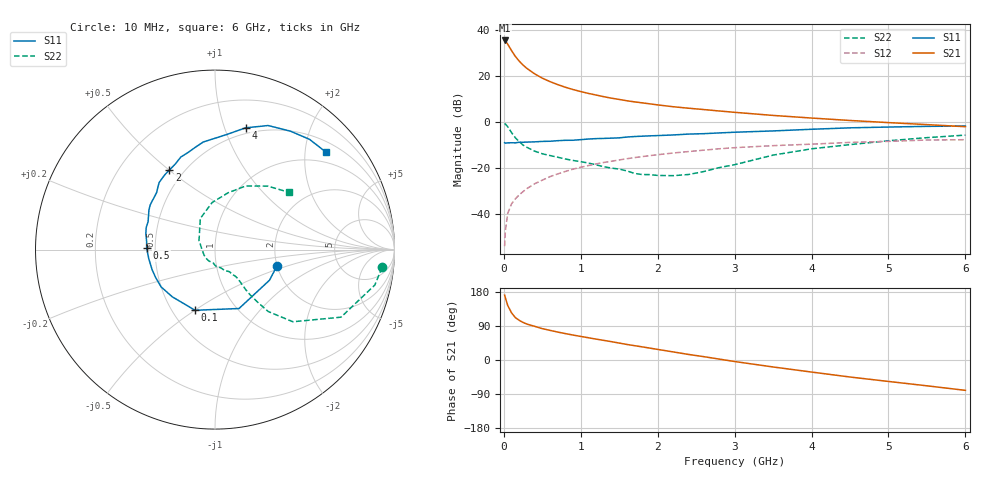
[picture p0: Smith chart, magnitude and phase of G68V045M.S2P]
! SIEMENS Small Signal Semiconductors
! BFG193
! Si NPN RF Bipolar Junction Transistor in SOT223
! VCE = 8 V  IC = 45 mA
! Common Emitter S-Parameters:  August  1996
# GHz  S  MA  R  50
!  f  S11  S21  S12  S22
! GHz  MAG  ANG  MAG  ANG  MAG  ANG  MAG  ANG
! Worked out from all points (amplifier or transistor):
!   36 points, 10 MHz to 6 GHz, reference 50 ohm
!   highest |S21| = 35.6 dB at 10 MHz (marker M1)
!   |S21| within 3 dB of that: start of sweep to 74.97 MHz
!   unconditionally stable (mu >= 1): 488.8 MHz to 2.429 GHz
!   at 250 MHz: K = 0.88, MSG = 27.5 dB, |S12| = -30.2 dB
!   at 1.4 GHz: K = 1.04, MAG = 12.4 dB, |S12| = -17.0 dB
!   at 6 GHz: K = 0.89, MSG = 2.8 dB, |S12| = -7.6 dB
!   S11 on the Smith chart (normalised r, x): 10 MHz: 1.99, -0.42; 100 MHz: 0.65, -0.50; 500 MHz: 0.45, +0.01; 2 GHz: 0.42, +0.50; 4 GHz: 0.44, +1.18; 6 GHz: 0.74, +2.48
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0.01  0.3569 -14.9  59.93 171.2  0.002 86.9  0.9361 -6.1
0.02  0.3483 -29.3  57.92 164.2  0.0043 80.8  0.9121 -12.5
0.05  0.3545 -67.8  49.83 144.1  0.0103 72.4  0.7967 -28.2
0.1  0.3559 -108.2  36.11 124.5  0.0167 66.9  0.5917 -42.8
0.15  0.3547 -132.1  26.86 111.8  0.0215 64.4  0.4554 -49.3
0.2  0.3652 -145.3  21.3 104.7  0.0262 66.0  0.376 -51.0
0.25  0.3655 -154.8  17.43 99.1  0.0308 66.7  0.317 -52.2
0.3  0.3679 -162.4  14.76 94.8  0.0358 67.3  0.283 -52.5
0.4  0.3726 -172.3  11.26 88.8  0.0456 67.6  0.2338 -52.1
0.5  0.3808 178.7  9.051 82.8  0.0546 67.1  0.205 -51.8
0.6  0.3839 173.0  7.622 78.2  0.0652 66.2  0.1875 -52.5
0.8  0.4025 162.3  5.738 69.7  0.0846 63.6  0.1576 -55.8
1.1  0.4291 149.1  4.218 58.7  0.1136 58.6  0.1288 -65.2
1.6  0.474 132.0  2.917 41.0  0.1601 48.2  0.0869 -90.5
2  0.5105 119.9  2.372 27.9  0.1956 39.3  0.0692 -132.4
2.2  0.526 114.8  2.167 21.4  0.2129 34.8  0.0684 -150.6
2.8  0.5827 100.4  1.75 2.4  0.2632 21.0  0.1026 150.4
3.5  0.6439 84.3  1.4 -18.4  0.3078 3.9  0.1916 115.3
4  0.6995 75.9  1.228 -31.8  0.3317 -5.8  0.2629 93.5
4.5  0.7521 66.8  1.087 -44.9  0.3625 -15.9  0.3244 77.1
5.5  0.8092 49.4  0.884 -68.1  0.4082 -39.1  0.4599 50.3
6  0.8234 41.1  0.796 -80.1  0.415 -52.5  0.5222 37.6
